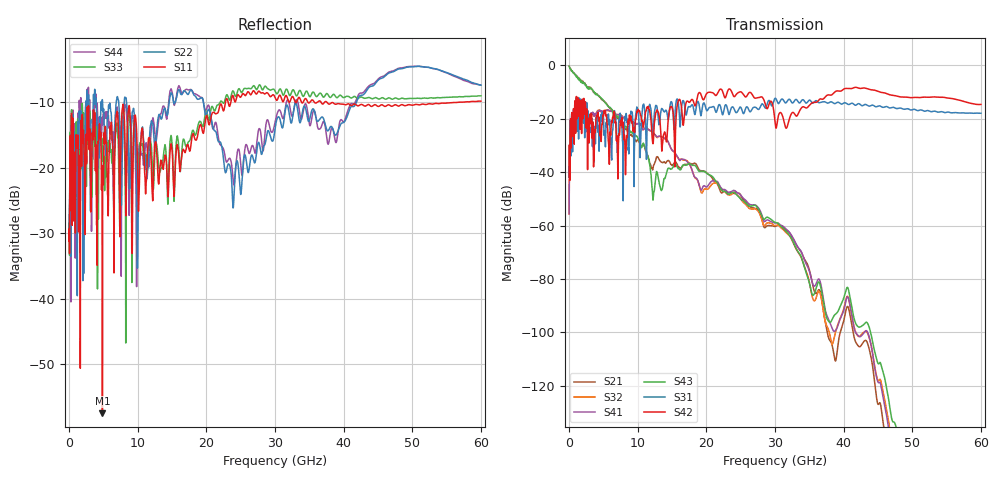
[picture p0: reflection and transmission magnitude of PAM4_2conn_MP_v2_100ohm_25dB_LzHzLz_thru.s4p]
! Info: Touchstone file created by Circ.  Input file=FAB50GbE_2conn_Midplane_Examax_Topo2_v2_100ohm_25dB_LzHzLz.circ
# Hz S RI R 50
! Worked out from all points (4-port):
!   6000 points, 10 MHz to 60 GHz, reference 50 ohm
!   strongest paths, dB at 10 MHz, 15.01 GHz, 30.01 GHz, 45.01 GHz, 60 GHz:
!     S42: -41.8, -15.8, -21.2, -9.7, -14.6
!     S31: -41.8, -14.3, -12.3, -15.2, -17.9
!     S43: -0.3, -38.6, -58.8, -111.5, -170.4
!     S41: -55.6, -31.7, -59.0, -118.6, -177.2
!     S32: -55.6, -31.7, -60.0, -118.0, -172.5
!     S21: -0.3, -37.5, -60.3, -126.9, -178.2
!   lowest |S11| = -57.5 dB at 4.86 GHz (marker M1), VSWR 1.00, Z = 49.9 + j0.0612 ohm
!   |S11| at or under -10 dB: start of sweep to 22.79 GHz; 36.7 GHz to 37.23 GHz (531.9 MHz wide, 1.44 % of centre); 37.55 GHz to 57.42 GHz (19.87 GHz wide, 41.8 % of centre)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
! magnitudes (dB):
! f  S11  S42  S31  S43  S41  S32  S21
! 10 MHz  -31.2  -41.8  -41.8  -0.3  -55.6  -55.6  -0.3
! 1 GHz  -15.4  -16.1  -17.5  -3.9  -18.4  -18.4  -3.8
! 4.86 GHz  -57.5  -21.7  -17.9  -12.7  -17.1  -17.4  -13.1
! 12.28 GHz  -21.7  -28.5  -23.5  -49.1  -25.2  -25.1  -37.8
! 18.3 GHz  -15.5  -15.0  -18.3  -37.5  -41.8  -41.9  -36.6
! 35.08 GHz  -10.0  -14.8  -13.0  -82.1  -77.6  -82.1  -77.2
! 60 GHz  -9.9  -14.6  -17.9  -170.4  -177.2  -172.5  -178.2
